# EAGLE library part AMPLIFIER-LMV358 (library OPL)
Low-Voltage Rail-To-Rail Output Operational Amplifiers
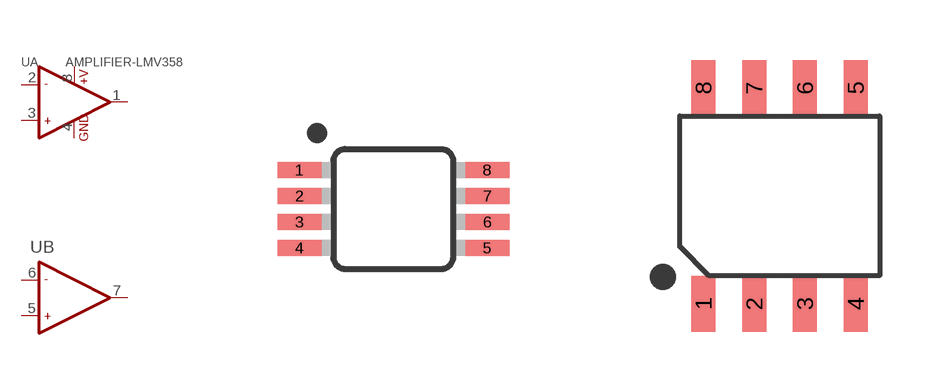
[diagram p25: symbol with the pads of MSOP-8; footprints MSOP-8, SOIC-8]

Designator prefix U; gates A=OPAMP_2-1 B=OPAMP_2_1-1

## AMPLIFIER-LMV358-310020007  [MSOP-8]
1  A:OUT1  out
2  A:-IN1  in
3  A:+IN1  in
4  A:GND  pwr
5  B:+IN2  in
6  B:-IN2  in
7  B:OUT2  out
8  A:+V  pwr

## AMPLIFIER-LMV358-310020002  [SOIC-8]
Pads as for MSOP-8

## Footprint MSOP-8 (pad centres in mm)
8M, 8-Lead, 0.118" Wide, Miniature Small Outline Package MSOP 8M-Package doc1097.pdf
smd 1.1 x 0.4: 1 -2.35,0.975; 2 -2.35,0.325; 3 -2.35,-0.325; 4 -2.35,-0.975; 5 2.35,-0.975; 6 2.35,-0.325; 7 2.35,0.325; 8 2.35,0.975

## Footprint SOIC-8 (pad centres in mm)
smd 0.6 x 1.4: 1 -1.905,-2.7; 2 -0.635,-2.7; 3 0.635,-2.7; 4 1.905,-2.7; 5 1.905,2.7; 6 0.635,2.7; 7 -0.635,2.7; 8 -1.905,2.7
